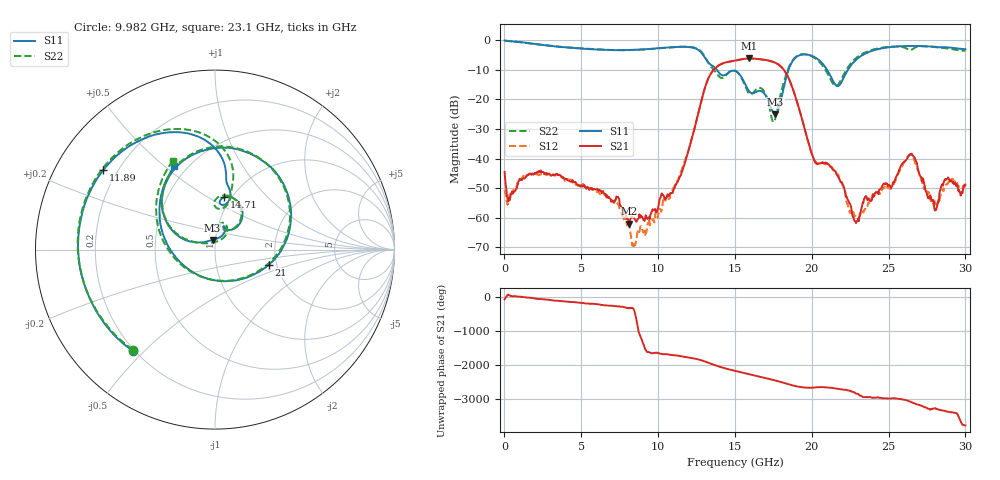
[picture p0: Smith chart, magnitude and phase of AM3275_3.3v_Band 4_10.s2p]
!Keysight Technologies,N5245B,MY58422270,A.16.20.02
!Date: Thursday, March 27, 2025 02:08:05
!Correction: S11(C  2-Port  )
!S21(C  2-Port  )
!S12(C  2-Port  )
!S22(C  2-Port  )
!S2P File: Measurements: S11, S21, S12, S22:
# Hz S  dB  R 50
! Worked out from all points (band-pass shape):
!   801 points, 10 MHz to 30 GHz, reference 50 ohm
!   highest |S21| = -6.22 dB at 15.94 GHz (marker M1); lowest = -62.0 dB at 8.107 GHz (marker M2)
!   |S21| within 3 dB of the highest: 13.78 GHz to 18.05 GHz (4.268 GHz wide, 26.8 % of centre)
!   lowest |S11| = -25.1 dB at 17.63 GHz (marker M3), VSWR 1.12, Z = 48.4 + j5.22 ohm
!   |S11| at or under -10 dB: 13.81 GHz to 18.49 GHz (4.679 GHz wide, 29 % of centre); 20.99 GHz to 22.36 GHz (1.373 GHz wide, 6.33 % of centre)
!   |S22| runs from -27.7 to -0.2 dB; largest |S21 - S12| = 0.0071
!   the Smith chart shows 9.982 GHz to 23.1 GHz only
!   S11 on the Smith chart (normalised r, x): 9.982 GHz: 0.19, -0.47; 11.89 GHz: 0.15, +0.31; 14.71 GHz: 0.93, +0.59; 21 GHz: 1.82, -0.34; 23.1 GHz: 0.43, +0.54
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1e7  -0.14 -3.6  -44.50 -77.1  -50.55 -178.1  -0.20 -4.7
1.2096e9  -0.80 -82.4  -46.76 -9.5  -45.95 -9.0  -0.83 -82.5
2.596638e9  -1.73 -161.5  -45.16 -81.6  -45.32 -78.8  -1.72 -161.3
5.033325e9  -2.90 89.5  -49.09 174.9  -48.75 177.0  -2.82 89.0
8.1073e9  -3.38 -42.3  -61.96 14.2  -61.70 -138.8  -3.41 -44.1
9.981675e9  -2.77 -128.7  -57.07 156.3  -60.00 131.5  -2.83 -129.4
1.001916e10  -2.76 -130.4  -56.13 140.5  -58.63 132.3  -2.81 -131.1
1.189354e10  -2.33 144.7  -38.81 23.3  -38.42 25.0  -2.24 144.9
1.365545e10  -9.14 76.9  -9.83 156.2  -9.84 156.1  -10.25 73.9
1.47051e10  -10.58 80.0  -7.22 17.0  -7.22 16.9  -10.52 84.9
1.5005e10  -10.42 67.9  -6.91 -15.9  -6.92 -15.9  -10.33 70.5
1.594219e10  -17.41 53.8  -6.22 -115.3  -6.22 -115.5  -18.16 61.2
1.669194e10  -17.20 67.2  -6.52 166.6  -6.51 166.5  -16.22 68.6
1.762912e10  -25.12 104.3  -7.68 62.3  -7.68 62.5  -26.46 129.8
1.867878e10  -7.77 136.3  -15.19 -74.3  -15.24 -74.4  -7.44 133.7
2.002832e10  -5.36 48.3  -38.80 -148.3  -38.77 -148.9  -5.57 45.2
2.1003e10  -10.11 -15.4  -41.53 -143.1  -42.15 -144.1  -11.10 -23.3
2.31023e10  -5.76 116.0  -59.59 -18.3  -59.65 -24.5  -5.23 115.2
2.501416e10  -2.46 50.5  -48.83 -105.0  -49.96 -109.5  -2.27 48.9
2.647618e10  -1.99 10.5  -38.42 146.5  -38.62 145.9  -3.30 12.5
2.748834e10  -2.11 -18.1  -51.94 -18.1  -51.21 -11.6  -2.19 -17.5
3e10  -3.10 -111.3  -48.78 -177.0  -49.57 -132.3  -3.59 -110.5
